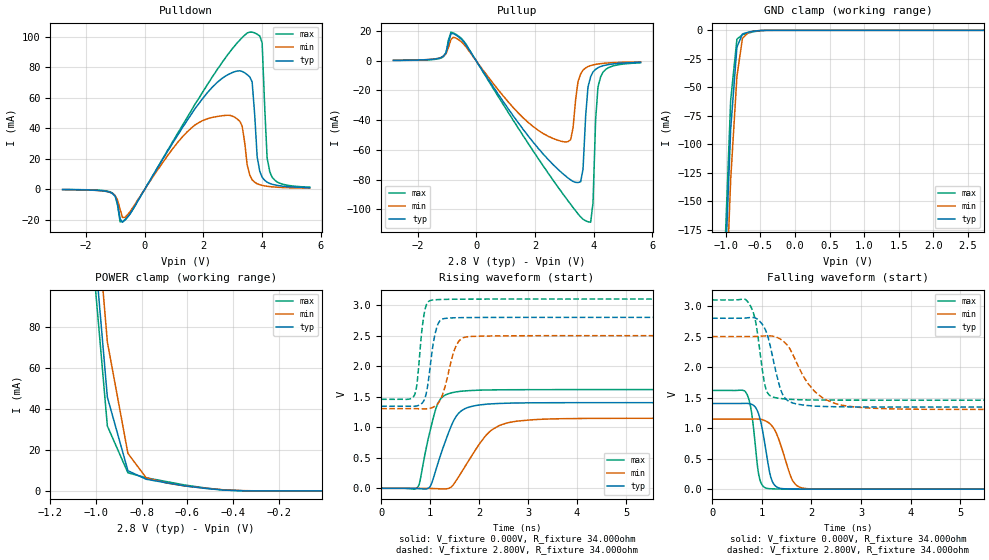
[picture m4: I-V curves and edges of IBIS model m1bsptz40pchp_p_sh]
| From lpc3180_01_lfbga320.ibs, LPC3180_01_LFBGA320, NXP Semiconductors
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| |   Rev 0.20 IBIS Model Design Automation Generation   |
| |   N O N - S I L I C O N   C O R R E L A T E D   |
| |   This IBIS [Model] is pre-Beta tactical support   |
| |  Note: this IBIS [Model] contains clamp curves generated   |
| |   through simulation which should not be relied upon   |
| mem1bsptz40pchp
|   Bidirectional Pad 2.8
|   3state Output
|   Plain Input
|   1ns Slew Rate control
|   CMOS
| Plain input Mode (p1=0, p2=1)
[Model]   m1bsptz40pchp_p_sh | of mem1bsptz40pchp
Model_type   I/O
Polarity   Non-Inverting
Enable   Active-Low
|  Reciever Thresholds
Vinl   = 0.36V
Vinh   = 0.84V
| AC Test Load Conditions
Vref   = 0
Cref   = 1.2e-11
Rref   = 1000000000
Vmeas   = 0.6
| [Process Range]   typical   min   max
| C_comp edge width   400.000ps   400.000ps   400.000ps
| C_comp Tstrobe   40.000fs   40.000fs   40.000fs
C_comp   2.023pF   1.952pF   2.111pF
[Temperature Range]   25   125   -40
[Voltage Range]   2.80V   2.50V   3.10V
[GND Clamp Reference]   0.00V   0.00V   0.00V
[Pulldown Reference]   0.00V   0.00V   0.00V
[POWER Clamp Reference]   2.80V   2.50V   3.10V
[Pullup Reference]   2.80V   2.50V   3.10V
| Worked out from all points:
|   slope of the pulldown table from 0 to 0.42 V, typ, clamps not added: 30.8 ohm
|   slope of the pullup table from 0 to 0.42 V, typ, clamps not added: 32.8 ohm
|   GND clamp passes 1 mA (typ) near -0.62 V on its own axis
|   POWER clamp passes 1 mA (typ) near -0.50 V on its own axis
|   rising waveform, V_fixture 0.000V, R_fixture 34.000ohm: 20-80 % time 380ps typ, 589ps min, 273ps max; typ from 0 V to 1.4 V
|   falling waveform, V_fixture 0.000V, R_fixture 34.000ohm: 20-80 % time 183ps typ, 282ps min, 135ps max; typ from 1.4 V to 0 V
|   rising waveform, V_fixture 2.800V, R_fixture 34.000ohm: 20-80 % time 156ps typ, 236ps min, 119ps max; typ from 1.34 V to 2.8 V
|   falling waveform, V_fixture 2.800V, R_fixture 34.000ohm: 20-80 % time 260ps typ, 554ps min, 175ps max; typ from 2.8 V to 1.34 V
[GND Clamp]
| ref voltage   0.00V   0.00V   0.00V
|   Voltage   I(typ)   I(min)   I(max)
-2.8V     -3.643A    -3.653A    -3.644A
-1.01V    -211.8mA   -255.9mA   -186.6mA
-930mV    -86.59mA   -130.6mA   -61.22mA
-840mV    -14.8mA    -40.63mA   -7.788mA
-760mV    -3.159mA   -7.066mA   -3.782mA
-670mV    -1.57mA    -1.656mA   -2.327mA
-500mV    -164.9uA   -160.9uA   -333.4uA
2.73V     191.3pA    5.77uA     169pA
[Power Clamp]   | Vtable = Vcc - Vpad
| ref voltage   2.80V   2.50V   3.10V
|   Voltage   I(typ)   I(min)   I(max)
-2.82V    3.531A     3.518A     3.546A
-1.03V    149.7mA    178.4mA    134.4mA
-950mV    45.7mA     72.61mA    31.64mA
-860mV    9.848mA    18.29mA    8.836mA
-780mV    5.694mA    6.392mA    6.4mA
-690mV    3.927mA    3.849mA    4.543mA
-610mV    2.433mA    2.409mA    2.865mA
-440mV    389uA      533.2uA    433.4uA
-350mV    49.46uA    132.2uA    33.93uA
-10mV     426.3pA    7.713nA    250.7pA
[Pulldown]
| ref voltage   0.00V   0.00V   0.00V
|   Voltage   I(typ)   I(min)   I(max)
-2.8V     -319.4uA   -345.4uA   -253.4uA
-1.18V    -2.16mA    -2.186mA   -1.788mA
-670mV    -20.32mA   -18.55mA   -19.96mA
2.13V     63.18mA    46.12mA    68.49mA
3.24V     77.6mA     44.48mA    97.75mA
3.58V     73.59mA    9.104mA    103mA
3.66V     70.25mA    6.083mA    103mA
3.83V     21.2mA     3.504mA    101.6mA
4V        7.749mA    2.422mA    96.02mA
4.17V     4.517mA    1.836mA    20.5mA
4.26V     3.724mA    1.635mA    11.42mA
5.62V     951.1uA    582.3uA    1.268mA
[Pullup]   | Vtable = Vcc - Vpad
| ref voltage   2.80V   2.50V   3.10V
|   Voltage   I(typ)   I(min)   I(max)
-2.82V    285.5uA    305.8uA    228.3uA
-520mV    14.78mA    13mA       15.38mA
2.79V     -73.2mA    -53.56mA   -85.24mA
3.22V     -80.21mA   -53.04mA   -96.65mA
3.47V     -82mA      -13.93mA   -103.2mA
3.64V     -72.97mA   -6.254mA   -106.7mA
3.81V     -17.59mA   -3.875mA   -108.5mA
3.9V      -10.76mA   -3.236mA   -108.7mA
3.98V     -7.521mA   -2.772mA   -95.82mA
4.07V     -5.763mA   -2.42mA    -39.47mA
4.24V     -3.891mA   -1.925mA   -10.83mA
5.6V      -1.047mA   -713.1uA   -1.374mA
[Ramp]
R_load   = 34.000ohm
|   dV/dt(typ)   dV/dt(min)   dV/dt(max)
dV/dt_r   972.249mV/345.000ps   809.371mV/540.000ps   1.110V/250.000ps
dV/dt_f   1.002V/240.000ps   841.020mV/470.000ps   1.124V/165.000ps
[Rising Waveform]  | cubic spline decimation from 2001 points
V_fixture   = 0.000V
R_fixture   = 34.000ohm
|   Time   V(typ)   V(min)   V(max)
0s        4.315nV    140.2nV    2.475nV
750ps     -4.658mV   315.4uV    23.48mV
995ps     24mV       -2.306mV   924.7mV
1.14ns    359mV      -6.116mV   1.355V
1.255ns   641.9mV    -10.58mV   1.498V
1.475ns   1.099V     60.1mV     1.571V
1.71ns    1.304V     353.3mV    1.595V
2.15ns    1.378V     874.5mV    1.61V
2.685ns   1.396V     1.089V     1.615V
10ns      1.403V     1.147V     1.617V
[Falling Waveform]  | cubic spline decimation from 2001 points
V_fixture   = 0.000V
R_fixture   = 34.000ohm
|   Time   V(typ)   V(min)   V(max)
0s        1.403V     1.147V     1.617V
710ps     1.405V     1.147V     1.544V
795ps     1.39V      1.149V     1.261V
940ps     1.226V     1.147V     238.9mV
1.11ns    507mV      1.104V     12.46mV
1.185ns   190.9mV    1.056V     6.921mV
1.28ns    50.33mV    940.9mV    3.752mV
1.615ns   2.778mV    153.2mV    674.2uV
1.85ns    986.4uV    13.88mV    274.1uV
10ns      126.4nV    388.9nV    82.77nV
[Rising Waveform]  | cubic spline decimation from 2001 points
V_fixture   = 2.800V
V_fixture_min = 2.500V
V_fixture_max = 3.100V
R_fixture   = 34.000ohm
|   Time   V(typ)   V(min)   V(max)
0s        1.345V     1.305V     1.458V
675ps     1.344V     1.305V     1.518V
735ps     1.351V     1.304V     1.733V
830ps     1.391V     1.302V     2.573V
890ps     1.467V     1.301V     2.906V
1.045ns   2.271V     1.323V     3.084V
1.205ns   2.748V     1.444V     3.093V
1.525ns   2.794V     2.324V     3.097V
1.74ns    2.797V     2.48V      3.098V
10ns      2.8V       2.5V       3.1V
[Falling Waveform]  | cubic spline decimation from 2001 points
V_fixture   = 2.800V
V_fixture_min = 2.500V
V_fixture_max = 3.100V
R_fixture   = 34.000ohm
|   Time   V(typ)   V(min)   V(max)
0s        2.8V       2.5V       3.1V
735ps     2.809V     2.5V       3.053V
870ps     2.805V     2.502V     2.774V
1.085ns   2.591V     2.51V      1.643V
1.285ns   1.925V     2.494V     1.497V
1.42ns    1.555V     2.433V     1.481V
1.55ns    1.438V     2.321V     1.472V
2.045ns   1.362V     1.62V      1.461V
2.615ns   1.349V     1.376V     1.459V
10ns      1.345V     1.305V     1.458V
